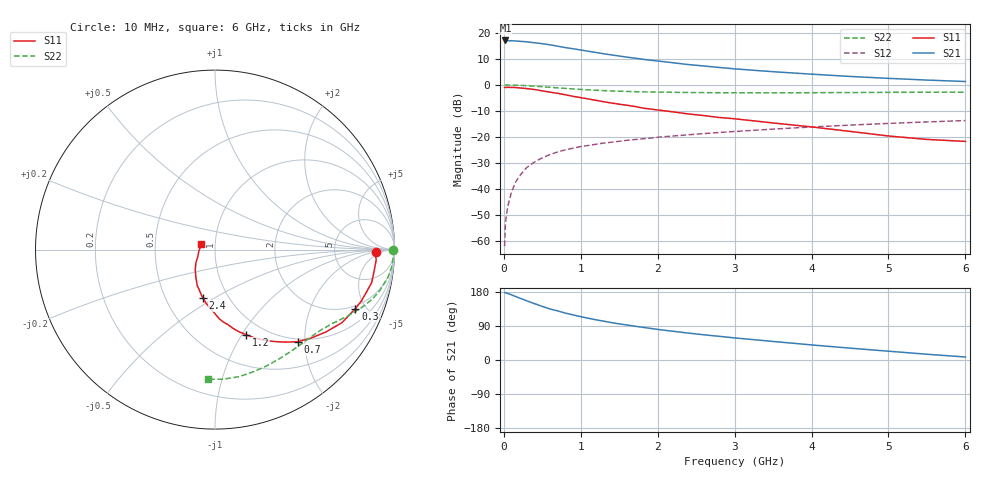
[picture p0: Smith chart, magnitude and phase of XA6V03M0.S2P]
! SIEMENS Discrete & RF Semiconductors
! BFY180
! Si NPN RF Bipolar Junction Transistor in MICRO-X
! VCE = 6 V  IC = 3 mA
! Common Emitter S-Parameters:  May  1997
# GHz  S  MA  R  50
!  f  S11  S21  S12  S22
! GHz  MAG  ANG  MAG  ANG  MAG  ANG  MAG  ANG
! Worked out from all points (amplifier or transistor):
!   36 points, 10 MHz to 6 GHz, reference 50 ohm
!   highest |S21| = 17.1 dB at 20 MHz (marker M1)
!   |S21| within 3 dB of that: start of sweep to 857 MHz
!   unconditionally stable (mu >= 1): 2.54 GHz to end of sweep
!   at 250 MHz: K = 0.14, MSG = 25.0 dB, |S12| = -33.3 dB
!   at 1.4 GHz: K = 0.76, MSG = 16.8 dB, |S12| = -22.0 dB
!   at 6 GHz: K = 1.05, MAG = 6.1 dB, |S12| = -13.7 dB
!   S11 on the Smith chart (normalised r, x): 10 MHz: 18, -2; 300 MHz: 1.80, -4.23; 700 MHz: 0.95, -1.85; 1.2 GHz: 0.82, -1.04; 2.4 GHz: 0.76, -0.44; 6 GHz: 0.86, +0.06
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0.01  0.8978 -0.8  7.14 178.1  0.0008 94.2  0.9927 -0.2
0.02  0.8934 -1.7  7.144 177.5  0.0022 94.8  0.9999 -0.6
0.05  0.9 -3.6  7.03 175.8  0.0046 84.9  0.9939 -1.9
0.1  0.8944 -7.9  7.069 171.9  0.0088 86.8  0.9915 -3.8
0.2  0.8763 -15.7  6.909 163.8  0.0174 81.0  0.9826 -7.4
0.3  0.8485 -22.8  6.719 155.9  0.0261 76.5  0.9651 -10.8
0.5  0.7698 -36.6  6.198 141.4  0.0398 68.6  0.9232 -16.9
0.6  0.7265 -42.8  5.889 134.6  0.0458 65.7  0.8997 -19.4
0.7  0.6896 -48.1  5.542 129.6  0.0517 62.3  0.8774 -21.7
0.8  0.6455 -53.0  5.205 123.7  0.0566 60.6  0.8561 -23.6
1  0.5687 -62.1  4.686 114.3  0.0655 56.7  0.82 -27.2
1.1  0.5375 -66.1  4.422 110.1  0.0688 55.0  0.8039 -28.7
1.2  0.5046 -69.9  4.197 106.0  0.0726 53.7  0.7907 -30.3
1.4  0.449 -77.2  3.769 98.6  0.0793 51.4  0.7663 -33.0
1.7  0.3859 -86.5  3.274 89.3  0.0891 49.1  0.7421 -36.9
2.2  0.3037 -99.3  2.664 75.8  0.1045 45.4  0.7209 -43.3
2.4  0.277 -104.3  2.458 71.0  0.1102 44.3  0.7152 -45.8
3  0.2238 -116.3  2.035 58.3  0.1276 40.3  0.7074 -53.1
3.5  0.186 -125.1  1.793 48.9  0.1417 37.1  0.7059 -59.3
4.5  0.1281 -145.9  1.455 31.3  0.169 30.1  0.7134 -72.3
5.5  0.0899 -175.2  1.239 15.2  0.1946 22.4  0.7234 -86.2
6  0.0822 157.0  1.163 7.9  0.2068 18.2  0.7245 -93.3
